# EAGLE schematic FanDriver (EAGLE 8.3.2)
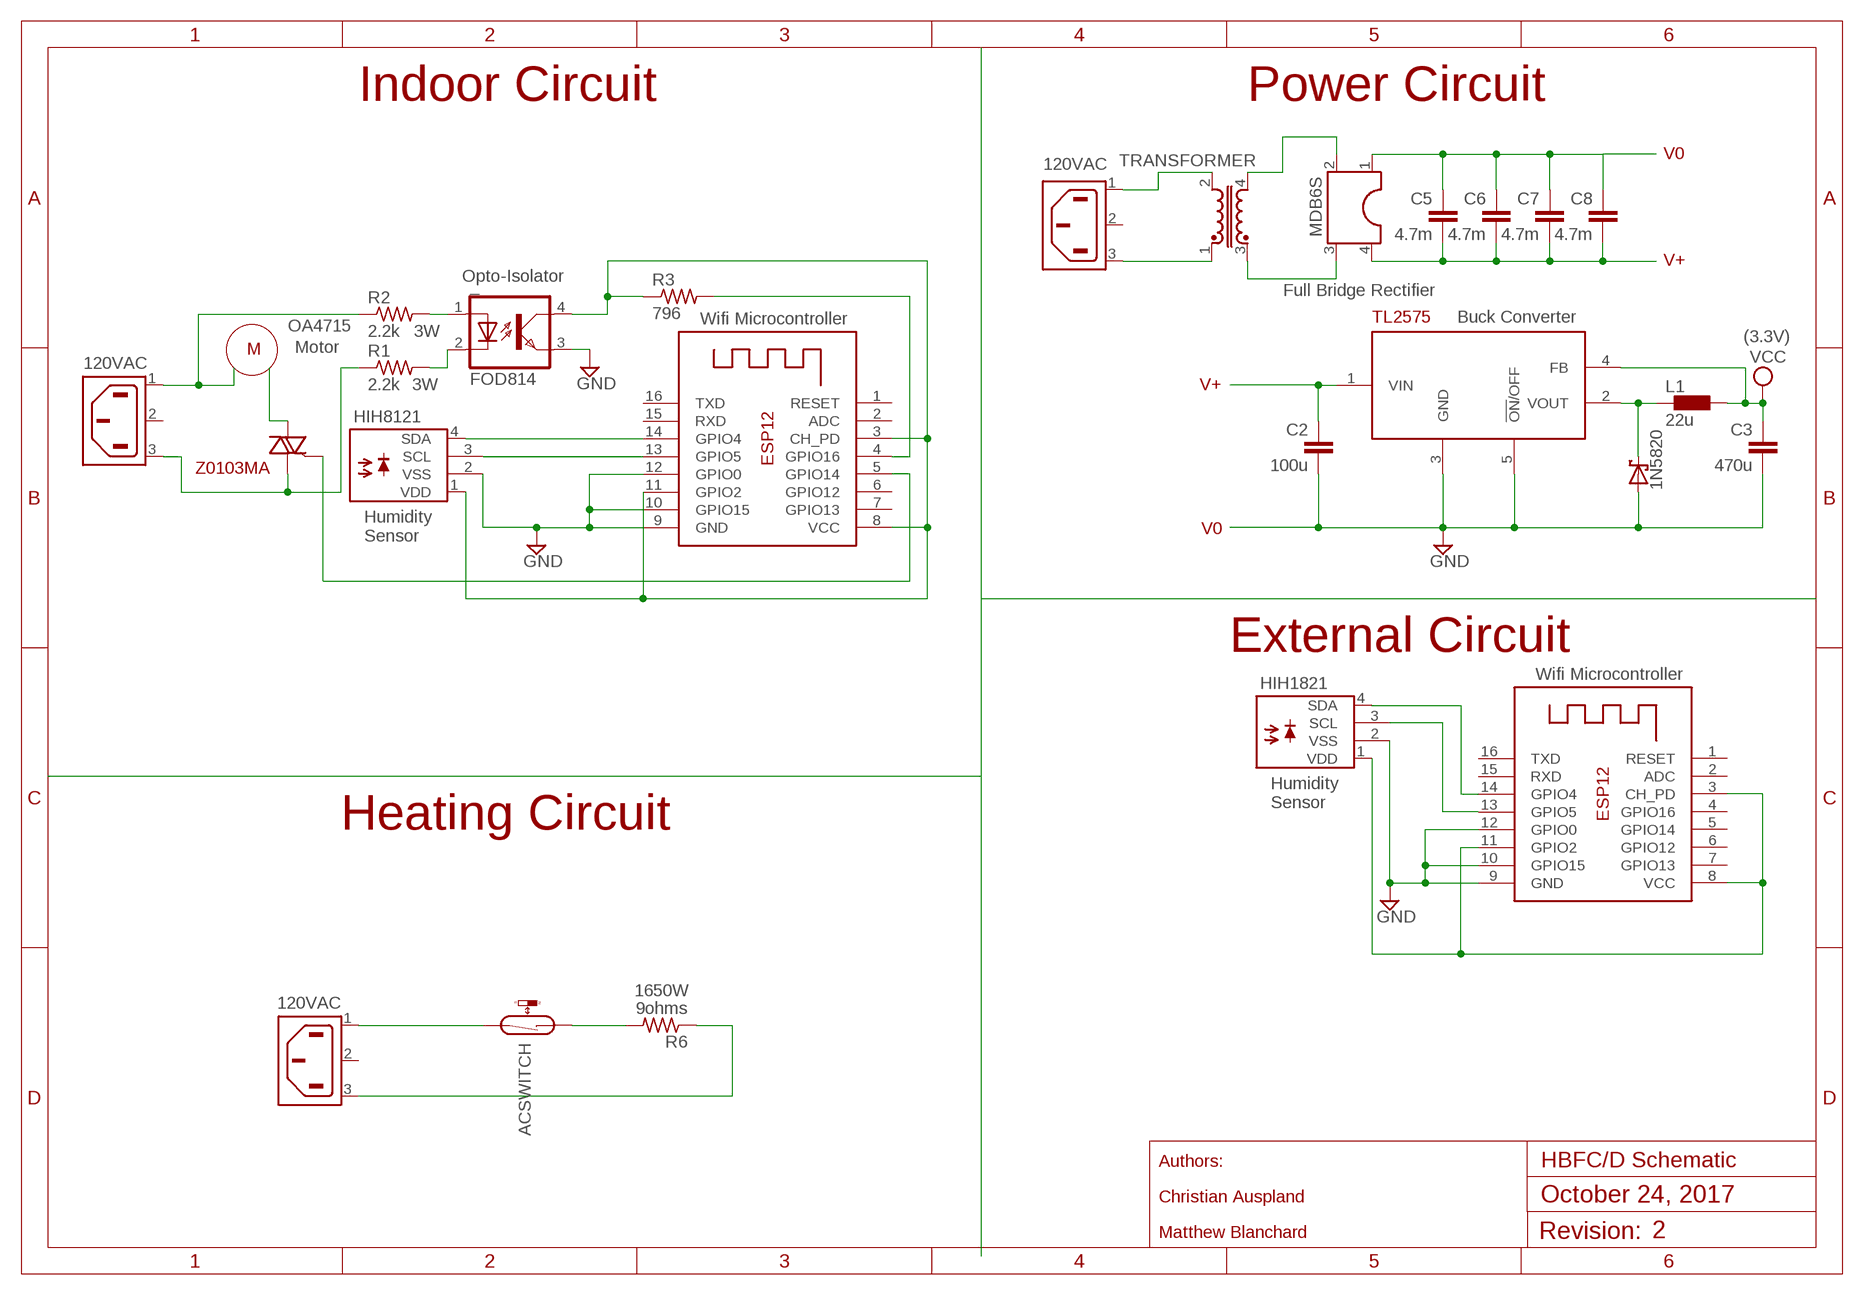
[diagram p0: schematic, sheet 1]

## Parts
_  FOD814  SFH618A-3  [DIP4]
C2  100u  C-EU025-024X044  [C025-024X044]
C3  470u  C-EU025-024X044  [C025-024X044]
C5  4.7m  C-EU025-024X044  [C025-024X044]
C6  4.7m  C-EU025-024X044  [C025-024X044]
C7  4.7m  C-EU025-024X044  [C025-024X044]
C8  4.7m  C-EU025-024X044  [C025-024X044]
HIH1821  HIH8121  [TO18PL4]
HIH8121  HIH8121  [TO18PL4]
L1  22u  L  [L1812]
R1  2.2k  R-US_MELF0102W  [MINI_MELF-0102W]
R2  2.2k  R-US_MELF0102W  [MINI_MELF-0102W]
R3  796  R-US_MELF0102W  [MINI_MELF-0102W]
R6  9ohms  R-US_MELF0102W  [MINI_MELF-0102W]
U$1  Z0103MA  [TO220BH]
U$6  ACSWITCH  [MK6-4]
U$7  TL2575  MYTL2575  [MYTL2575]
U$8  TRANSFORMER  [TRANSFORMER]
U$9  MDB6S  [MDB6S]
U$13  1N5820  [1N5820]
X1  ESP-12  [ESP-12]
X2  6ESRM-P  [6ESRM-P]
X3  6ESRM-P  [6ESRM-P]
X4  6ESRM-P  [6ESRM-P]
X5  ESP-12  [ESP-12]

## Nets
GND: _.3(EMIT) C2.2 C3.2 HIH1821.2(VSS) HIH8121.2(VSS) U$7.3(GND) U$7.5(!ON!/OFF) U$13.A X1.9(GND) X1.10(GPIO15) X1.12(GPIO0) X5.9(GND) X5.10(GPIO15) X5.12(GPIO0)
N$1: U$6.2 X3.1(AC1)
N$2: R2.1 X2.1(AC1)
N$3: U$1.T1(A2)
N$4: _.2(C) R1.2
N$5: _.1(A) R2.2
N$6: R1.1 U$1.G(A1) X2.3(AC2)
N$7: U$1.T2(G) X1.5(GPIO14)
N$8: HIH8121.3(SCL) X1.13(GPIO5)
N$9: R3.2 X1.4(GPIO16)
N$10: HIH8121.4(SDA) X1.14(GPIO4)
N$12: R6.2 U$6.1
N$13: R6.1 X3.3(AC2)
N$15: U$8.2 X4.1(AC1)
N$16: U$8.4 U$9.2
N$17: C2.1 U$7.1(VIN)
N$18: U$8.3 U$9.3
N$19: L1.2 U$7.2(VOUT) U$13.C
N$20: C5.2 C6.2 C7.2 C8.2 U$9.4
N$21: _.4(COL) HIH8121.1(VDD) R3.1 X1.3(CH_PD) X1.8(VCC) X1.11(GPIO2)
N$22: C5.1 C6.1 C7.1 C8.1 U$9.1
N$23: U$8.1 X4.3(AC2)
N$24: HIH1821.4(SDA) X5.14(GPIO4)
N$25: HIH1821.3(SCL) X5.13(GPIO5)
N$26: HIH1821.1(VDD) X5.3(CH_PD) X5.8(VCC) X5.11(GPIO2)
VCC: C3.1 L1.1 U$7.4(FB)
Unconnected: X1.1(RESET) X1.2(ADC) X1.6(GPIO12) X1.7(GPIO13) X1.15(RXD) X1.16(TXD) X2.2(SH) X3.2(SH) X4.2(SH) X5.1(RESET) X5.2(ADC) X5.4(GPIO16) X5.5(GPIO14) X5.6(GPIO12) X5.7(GPIO13) X5.15(RXD) X5.16(TXD)

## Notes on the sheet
- Indoor Circuit | Power Circuit
- V0
- 120VAC
- V+
- Opto-Isolator
- Full Bridge Rectifier
- Wifi Microcontroller | Buck Converter
- OA4715
- 3W
- (3.3V)
- M | Motor
- 120VAC
- 3W | V+
- V0
- Humidity
  Sensor
- External Circuit
- Wifi Microcontroller
- Humidity
  Sensor
- Heating Circuit
- 1650W
- 120VAC

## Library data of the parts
_ = optocoupler:SFH618?*: Optocoupler, Phototransistor Output, Low Input Current Source: Data sheet; MF: VISHAY/TELEFUNKEN; MPN: SFH618A-3; OC_FARNELL: 1020374; OC_NEWARK: 58K2209
C2 C3 C5-C8 = resistor:C-EU: CAPACITOR, European symbol
HIH1821 HIH8121 = MyLibrary:HIH8121
L1 = eagle-ltspice:L: INDUCTOR, European symbol; SPICEMODEL: NONE; SPICEPREFIX: L
R1-R3 R6 = adafruit:R-US_: RESISTOR, American symbol
U$1 = MyLibrary:Z0103MA
U$6 = MyLibrary:ACSWITCH
U$7 = MyLibrary:MYTL2575
U$8 = MyLibrary:TRANSFORMER
U$9 = MyLibrary:MDB6S
U$13 = MyLibrary:1N5820
X1 X5 = adafruit:ESP-12
X2-X4 = con-tycoelectronics:6ESRM-P: AC Connector 120/250 VAC Source: http://catalog.tycoelectronics.com .. ENG_DS_1654001_1099_SR_0406.pdf; MF: TYCO ELECTRONICS; MPN: 6ESRM-P; OC_FARNELL: unknown; OC_NEWARK: 87F1821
